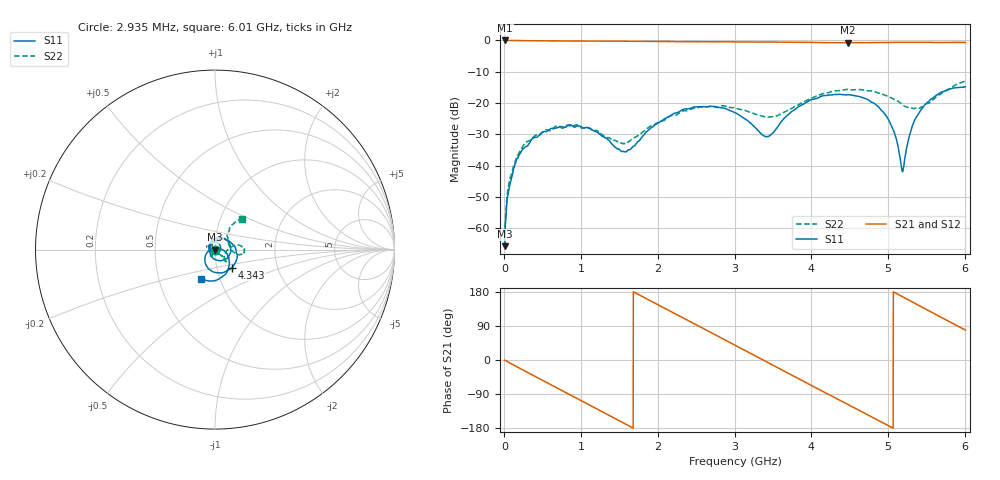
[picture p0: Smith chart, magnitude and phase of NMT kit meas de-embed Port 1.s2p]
! Carlisle Launcher - Use on Port1  07/02/2020  12:31:25
! Ref Plane: 0.000 mm
# MHZ S MA R  50
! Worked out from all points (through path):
!   2048 points, 2.935 MHz to 6.01 GHz, reference 50 ohm
!   highest |S21| = 0.00 dB at 8.804 MHz (marker M1); lowest = -0.7 dB at 4.478 GHz (marker M2)
!   group delay of S21, straight-line fit = 296 ps
!   lowest |S11| = -65.7 dB at 2.935 MHz (marker M3), VSWR 1.00, Z = 50 - j0.0318 ohm
!   |S11| at or under -10 dB: start of sweep to end of sweep
!   |S22| runs from -64.7 to -13.0 dB; largest |S21 - S12| = 0.0063
!   S11 on the Smith chart (normalised r, x): 2.935 MHz: 1.00, -0.00; 4.343 GHz: 1.18, -0.24; 6.01 GHz: 0.82, -0.28
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2.9346  0.00052 -37.6  0.9995 -0.4  0.9994 -0.3  0.00058 -24.9
8.8037  0.00086 -58.3  0.9995 -1.0  0.9992 -1.0  0.00103 -52.8
44.0186  0.00343 -94.8  0.998 -4.9  0.9981 -4.9  0.004 -70.3
79.2334  0.00548 -103.6  0.997 -8.7  0.9971 -8.8  0.00658 -73.9
264.1113  0.01941 -141.0  0.9919 -28.7  0.9918 -28.7  0.02243 -95.3
648.54  0.03993 150.1  0.9834 -69.8  0.983 -69.9  0.04053 -120.0
1006.558  0.04155 75.9  0.9773 -107.9  0.9771 -107.9  0.03994 -123.2
1567.06  0.0167 -98.0  0.9721 -167.8  0.9722 -167.8  0.02273 -79.7
2007.246  0.04838 121.8  0.963 145.3  0.9631 145.3  0.04953 -42.5
2511.992  0.08742 27.0  0.9542 91.8  0.9548 91.7  0.08399 -45.7
3007.934  0.07015 -61.8  0.9478 38.9  0.9486 38.8  0.08378 -49.6
3427.578  0.02915 166.6  0.9421 -5.8  0.9423 -5.9  0.0596 -26.0
4008.623  0.1139 5.0  0.9297 -67.8  0.932 -67.9  0.1202 11.2
4343.164  0.1373 -47.0  0.9198 -103.2  0.9215 -103.1  0.1577 5.0
4478.154  0.1359 -67.5  0.918 -117.3  0.9209 -117.2  0.165 0.7
4821.498  0.09863 -121.0  0.9242 -153.5  0.9234 -153.5  0.1524 -9.7
5009.311  0.05375 -154.8  0.9291 -173.5  0.9298 -173.5  0.126 -10.9
5191.254  0.00802 92.0  0.931 166.8  0.9335 166.8  0.09426 -4.3
5320.375  0.04391 -2.4  0.9328 153.0  0.936 152.9  0.08275 12.9
5461.235  0.08737 -29.8  0.933 137.7  0.9369 137.6  0.08868 36.3
5728.281  0.1536 -72.4  0.9295 109.0  0.9337 108.8  0.1528 56.0
6009.999  0.1818 -114.7  0.9309 79.0  0.9335 78.8  0.2247 48.8
